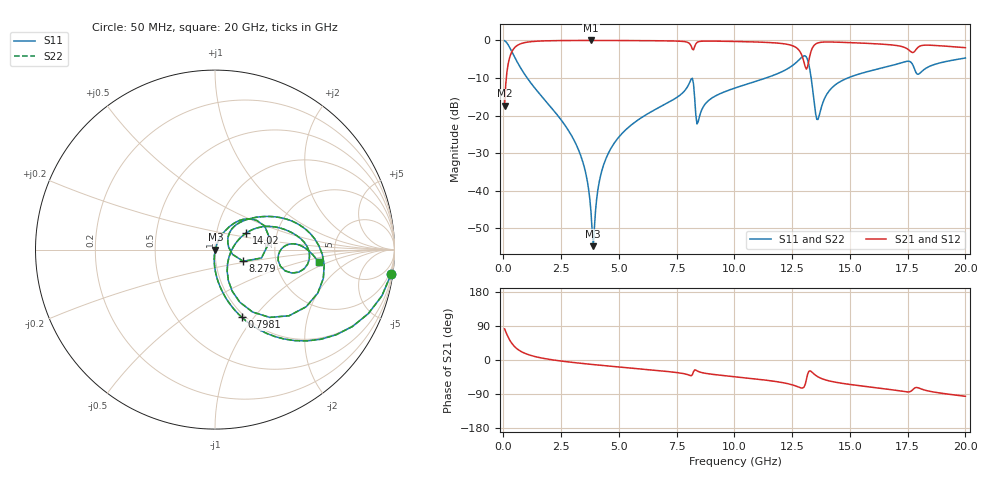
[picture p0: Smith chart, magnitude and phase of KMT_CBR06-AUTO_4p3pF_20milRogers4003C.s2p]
! Data measured by Modelithics Inc. support@modelithics.com 813-866-6335
! KEMET CBR06-AUTO 4.3pF, Pad Width= 0.851mm, Pad Length= 0.64mm, Pad Gap= 0.62mm, 20mil Rogers 4003C substrate Data, January 2022
# hz S ma R 50
! 2 Port Network Data from SP1.SP block
! freq  magS11  angS11  magS21  angS21  magS12  angS12  magS22  angS22
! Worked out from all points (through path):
!   401 points, 50 MHz to 20 GHz, reference 50 ohm
!   highest |S21| = -0.02 dB at 3.791 GHz (marker M1); lowest = -17.4 dB at 50 MHz (marker M2)
!   group delay of S21, straight-line fit = 15.3 ps
!   lowest |S11| = -54.8 dB at 3.89 GHz (marker M3), VSWR 1.00, Z = 50.2 - j0.0125 ohm
!   |S11| at or under -10 dB: 1.027 GHz to 11.37 GHz (10.34 GHz wide, 167 % of centre); 13.32 GHz to 14.91 GHz (1.589 GHz wide, 11.3 % of centre)
!   |S22| runs from -54.8 to -0.1 dB; largest |S21 - S12| = 0
!   S11 on the Smith chart (normalised r, x): 50 MHz: 1, -14; 798.1 MHz: 0.96, -0.87; 8.279 GHz: 1.36, -0.18; 14.02 GHz: 1.39, +0.26; 20 GHz: 3.61, -0.78
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5e7  0.9908 -7.9  0.1349 82.1  0.1349 82.1  0.9908 -7.9
2.99375e8  0.773 -40.2  0.6336 49.7  0.6336 49.7  0.773 -40.2
7.98125e8  0.4036 -68.5  0.9139 21.3  0.9139 21.3  0.4036 -68.5
3.391625e9  0.02662 -95.4  0.9978 -9.0  0.9978 -9.0  0.02662 -95.4
3.790625e9  0.005166 -81.3  0.9981 -11.5  0.9981 -11.5  0.005166 -81.3
3.890375e9  0.001822 -3.9  0.9981 -12.1  0.9981 -12.1  0.001822 -3.9
4.189625e9  0.0151 69.0  0.9979 -13.8  0.9979 -13.8  0.0151 69.0
4.6385e9  0.03583 70.4  0.9972 -16.4  0.9972 -16.4  0.03583 70.4
6.73325e9  0.1279 60.5  0.9886 -28.1  0.9886 -28.1  0.1279 60.5
8.12975e9  0.3065 25.4  0.8386 -41.4  0.8386 -41.4  0.3065 25.4
8.279375e9  0.17 -22.6  0.83 -26.1  0.83 -26.1  0.17 -22.6
8.429e9  0.08222 30.2  0.9564 -30.1  0.9564 -30.1  0.08222 30.2
1.0025e10  0.2323 44.6  0.9676 -44.2  0.9676 -44.2  0.2323 44.6
1.2419e10  0.4416 22.1  0.8682 -64.1  0.8682 -64.1  0.4416 22.1
1.296762e10  0.6146 -8.1  0.5739 -73.6  0.5739 -73.6  0.6146 -8.1
1.316712e10  0.5532 -41.8  0.4468 -38.2  0.4468 -38.2  0.5532 -41.8
1.336662e10  0.2505 -67.5  0.784 -32.5  0.784 -32.5  0.2505 -67.5
1.3616e10  0.08858 -9.8  0.9253 -44.4  0.9253 -44.4  0.08858 -9.8
1.4015e10  0.1952 27.9  0.9525 -53.8  0.9525 -53.8  0.1952 27.9
1.670825e10  0.4545 10.6  0.8761 -77.6  0.8761 -77.6  0.4545 10.6
1.770575e10  0.4834 -15.0  0.6899 -79.4  0.6899 -79.4  0.4834 -15.0
2e10  0.5826 -7.1  0.7995 -95.8  0.7995 -95.8  0.5826 -7.1
